(* Logix 5000 AddOnInstructionDefinition export AMCI_3601_AOP_Resume; software revision 20.03 *)

ADD_ON_INSTRUCTION AMCI_3601_AOP_Resume   (* revision 0.0, vendor AMCI, ExecuteEnableInFalse *)
// Revision note:
// 3/2020: Version 0 is the initial release
VAR_INPUT
   Axis_Status_Bits : INT; {required}
END_VAR
VAR_OUTPUT
   EN : BOOL; {access Read Only, visible}
   ER : BOOL; {access Read Only, visible}
END_VAR
VAR_IN_OUT
   AMCI_3601_output_data : AM:1769_3601:O:0; {required}
END_VAR
VAR
   Upper_Result_X_1000 : DINT;
   command_data_block : INT[10];
        [0]   // Command Bits MSW
        [1]   // Command Bits LSW
        [2]   // Upper Target Position
        [3]   // Lower Target Position
        [4]   // Upper Programmed Speed
        [5]   // Lower Programmed Speed
END_VAR

ROUTINE EnableInFalse   (* ladder *)
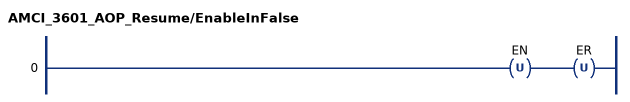
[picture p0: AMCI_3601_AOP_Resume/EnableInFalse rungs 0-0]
   0: OTU(EN)OTU(ER);
END_ROUTINE

ROUTINE Logic   (* ladder *)
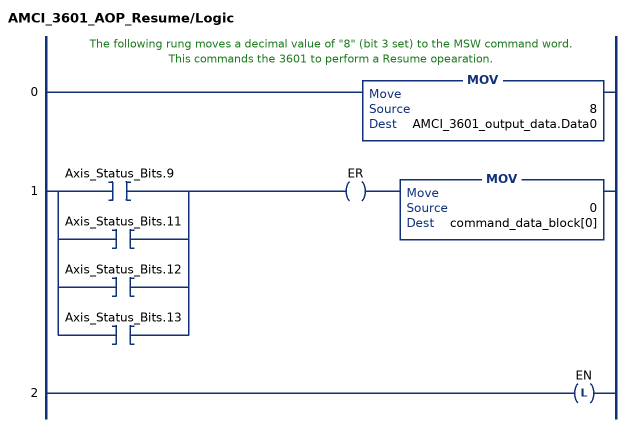
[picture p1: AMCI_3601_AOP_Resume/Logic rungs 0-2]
   // The following rung moves a decimal value of "8" (bit 3 set) to the MSW command word.  This commands the 3601 to perform a Resume opearation.
   0: MOV(8,AMCI_3601_output_data.Data0);
   1: [XIC(Axis_Status_Bits.9) ,XIC(Axis_Status_Bits.11) ,XIC(Axis_Status_Bits.12) ,XIC(Axis_Status_Bits.13) ]OTE(ER)MOV(0,command_data_block[0]);
   2: OTL(EN);
END_ROUTINE
END_ADD_ON_INSTRUCTION
